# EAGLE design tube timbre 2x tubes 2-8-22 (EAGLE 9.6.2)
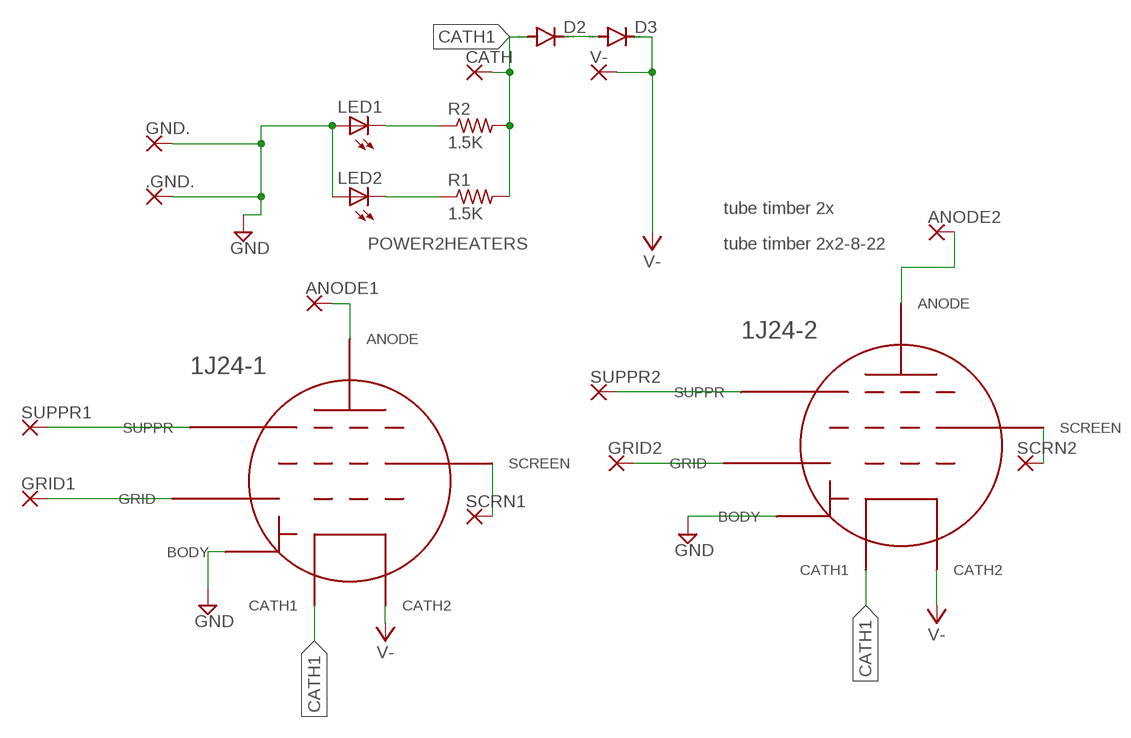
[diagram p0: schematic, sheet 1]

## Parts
1J24-1  1J24B  [6PINSOLDER]
1J24-2  1J24B  [6PINSOLDER]
.GND.  1  WIREPAD1,6/0,9  [1,6/0,9]
ANODE1  1  WIREPAD2,54/1,0  [2,54/1,0]
ANODE2  1  WIREPAD2,54/1,0  [2,54/1,0]
CATH  1  WIREPAD1,6/0,9  [1,6/0,9]
D2  1N4148DO35-7  [DO35-7]
D3  1N4148DO35-7  [DO35-7]
GND.  1  WIREPAD1,6/0,9  [1,6/0,9]
GRID1  1  WIREPAD1,6/0,9  [1,6/0,9]
GRID2  1  WIREPAD1,6/0,9  [1,6/0,9]
LED1  LED3MM  [LED3MM]
LED2  LED3MM  [LED3MM]
R1  1.5K  R-US_0207/10  [0207/10]
R2  1.5K  R-US_0207/10  [0207/10]
SCRN1  1  WIREPAD1,6/0,9  [1,6/0,9]
SCRN2  1  WIREPAD1,6/0,9  [1,6/0,9]
SUPPR1  1  WIREPAD1,6/0,9  [1,6/0,9]
SUPPR2  1  WIREPAD1,6/0,9  [1,6/0,9]
V-  1  WIREPAD1,6/0,9  [1,6/0,9]

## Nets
CATH1: 1J24-1.1-CATH(CATH1) 1J24-2.1-CATH(CATH1) CATH.1(P) D2.A R1.2 R2.2
GND: 1J24-1.3-BDY(BODY) 1J24-2.3-BDY(BODY) .GND..1(P) GND..1(P) LED1.A LED2.A
N$1: 1J24-2.6-GRID(GRID) GRID2.1(P)
N$2: 1J24-1.4-SUPP(SUPPR) SUPPR1.1(P)
N$3: LED2.K(C) R1.1
N$4: 1J24-1.6-GRID(GRID) GRID1.1(P)
N$5: LED1.K(C) R2.1
N$6: 1J24-1.5-SCR(SCREEN) SCRN1.1(P)
N$7: 1J24-2.4-SUPP(SUPPR) SUPPR2.1(P)
N$8: 1J24-1.A(ANODE) ANODE1.1(P)
N$9: D2.C D3.A
N$10: 1J24-2.A(ANODE) ANODE2.1(P)
N$11: 1J24-2.5-SCR(SCREEN) SCRN2.1(P)
V-: 1J24-1.2-CATH(CATH2) 1J24-2.2-CATH(CATH2) D3.C V-.1(P)

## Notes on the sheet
- tube timber 2x
- POWER2HEATERS | tube timber 2x2-8-22

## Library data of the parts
1J24-1 1J24-2 = submini tubes CL:1J24B
.GND. ANODE1 ANODE2 CATH GND. GRID1 GRID2 SCRN1 SCRN2 SUPPR1 SUPPR2 V- = wirepad:WIREPAD: Wire PAD connect wire on PCB; SPICEPREFIX: X
D2 D3 = diode:1N4148: DIODE; SPICEPREFIX: D
LED1 LED2 = adafruit:LED: LED; SPICEPREFIX: L
R1 R2 = resistor:R-US_: RESISTOR, American symbol; SPICEPREFIX: R

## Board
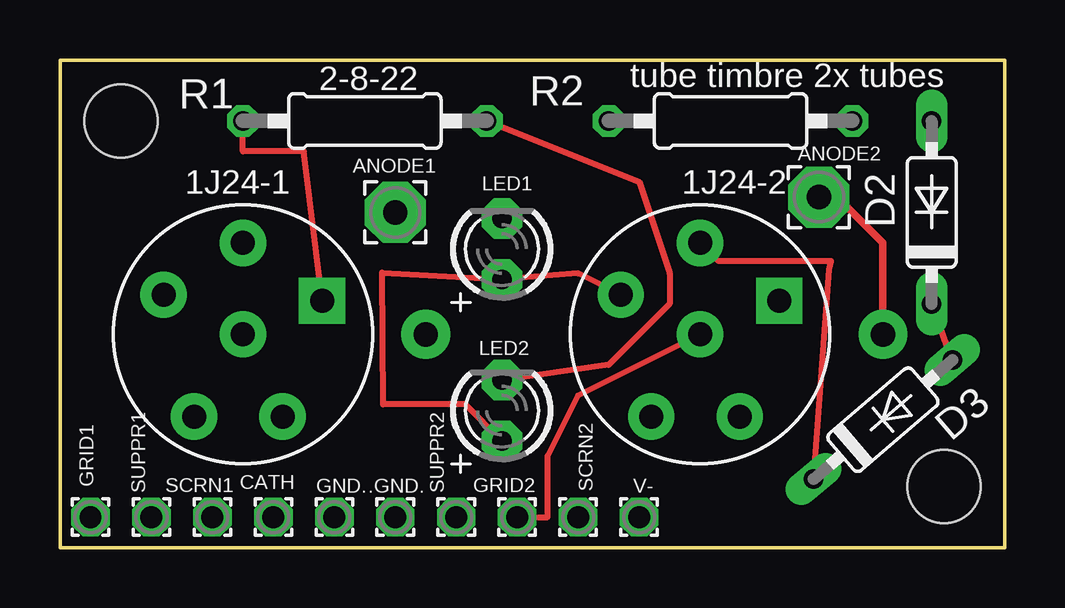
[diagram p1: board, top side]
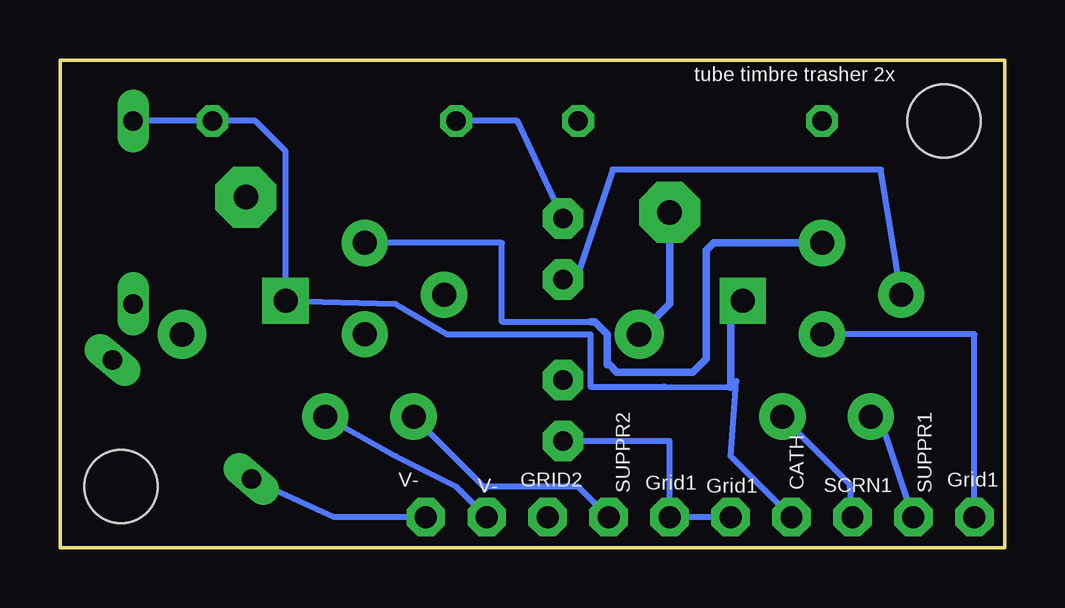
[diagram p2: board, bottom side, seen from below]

Size 39.37 x 20.32 mm. Coordinates in mm from the lower left corner, seen from the top.
Outline: 0,0 0,20.32 39.37,20.32 39.37,0 0,0
Copper layers (1*16): Top 0.035mm / dielectric 1.5mm / Bottom 0.035mm
Design rules "default": minimum track width 6mil, minimum drill 0.35mm, track to track 6mil, track to pad 6mil, pad to pad 6mil, via to via 6mil, smd to smd 6mil, copper to edge 40mil, drill to drill 6mil, minimum pad ring 10mil, minimum via ring 8mil, stop-mask expansion 4mil, vias tented up to drill 0mil, thermal gap 10mil
Holes 3.05 mm at 2.54,17.78 36.83,2.54

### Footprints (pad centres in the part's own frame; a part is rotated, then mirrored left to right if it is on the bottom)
6PINSOLDER = drill 1 pad 1.93 square: 1-CATH 5.842,2.667 | drill 1 pad 1.93: 2-CATH 2.54,5.08; 3-BDY -0.762,2.921; 4-SUPP 0.508,-2.159; 5-SCR 4.191,-2.159; 6-GRID 2.54,1.27 | drill 1.016 pad 2.032: A 10.16,1.27
1,6/0,9 = drill 0.914 pad 1.6 octagon: 1 0,0
2,54/1,0 = drill 1.016 pad 2.54 octagon: 1 0,0
DO35-7 = drill 0.813 long: A 3.81,0; C -3.81,0
LED3MM = drill 0.813 pad 1.676 octagon: A -1.27,0; K 1.27,0
0207/10 = drill 0.813 octagon: 1 -5.08,0; 2 5.08,0

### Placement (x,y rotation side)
1J24-1  5.08,7.62 0 top
1J24-2  24.13,7.62 0 top
.GND.  13.97,1.27 0 top
ANODE1  13.97,13.97 0 top
ANODE2  31.62,14.61 0 top
CATH  8.89,1.27 0 top
D2  36.32,13.97 90 top
D3  34.29,5.33 40.6 top
GND.  11.43,1.27 0 top
GRID1  1.27,1.27 0 top
GRID2  19.05,1.27 0 top
LED1  18.41,12.45 90 top
LED2  18.41,5.71 90 top
R1  12.7,17.78 180 top
R2  27.94,17.78 0 top
SCRN1  6.35,1.27 0 top
SCRN2  21.59,1.27 0 top
SUPPR1  3.81,1.27 0 top
SUPPR2  16.51,1.27 0 top
V-  24.13,1.27 0 top

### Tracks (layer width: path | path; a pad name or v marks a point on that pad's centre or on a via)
CATH1
  Top 0.254: 1J24-1.1-CATH 10.16,16.51 7.62,16.51 R1.2
  Bottom 0.254: D2.A R2.2 31.24,17.78 29.97,16.51 1J24-2.1-CATH 25.4,10.16 23.24,8.89 17.27,8.89 17.27,6.71 14.21,6.71 11.43,6.68 | CATH.1 11.43,3.81 11.19,6.94 11.43,6.94
  Bottom 0.305: 11.43,6.68 11.43,6.94 11.43,9.78 1J24-1.1-CATH
GND
  Top 0.254: 1J24-2.3-BDY 21.59,11.43 LED1.A 13.43,11.46 13.46,5.97 16.89,5.97 LED2.A
  Bottom 0.254: 1J24-1.3-BDY 5.16,15.75 16.34,15.75 17.78,11.43 LED1.A | GND..1 .GND..1 13.97,4.45 LED2.A
N$1
  Top 0.254: GRID2.1 20.32,1.27 20.32,3.81 21.59,6.35 1J24-2.6-GRID
N$2
  Bottom 0.254: SUPPR1.1 5.08,5.08 1J24-1.4-SUPP
N$3
  Top 0.254: R1.1 24.13,15.24 25.4,11.43 25.4,10.16 22.86,7.62 LED2.K
N$4
  Bottom 0.254: GRID1.1 1.27,8.89 1J24-1.6-GRID
N$5
  Bottom 0.254: LED1.K 20.32,17.78 R2.1
N$6
  Bottom 0.254: 1J24-1.5-SCR 6.48,2.67 SCRN1.1
N$7
  Bottom 0.254: SUPPR2.1 17.78,2.54 21.69,2.54 21.65,2.47 1J24-2.4-SUPP
N$8
  Bottom 0.305: 1J24-1.A 13.97,10.16 ANODE1.1
N$9
  Top 0.254: D3.A D2.C
N$10
  Top 0.305: 1J24-2.A 34.29,12.7 32.38,14.61 ANODE2.1
N$11
  Bottom 0.254: SCRN2.1 22.86,2.54 25.4,3.81 1J24-2.5-SCR
V-
  Top 0.254: D3.C 32.04,11.59 32.13,11.94 27.43,11.94 1J24-2.2-CATH
  Bottom 0.254: 17.25,9.42 20.95,9.42 20.95,12.7 1J24-2.2-CATH | V-.1 27.94,1.27 D3.C
  Bottom 0.305: 17.25,9.42 17.09,9.42 16.56,8.89 16.56,7.62 16.47,7.62 16.17,7.32 13.01,7.32 12.45,7.87 12.45,12.39 12.14,12.7 1J24-1.2-CATH

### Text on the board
tNames: 2-8-22 | tube timbre 2x tubes
bNames: tube timbre trasher 2x | Grid1 | SCRN1 | GRID2 | V- | SUPPR1 | CATH | Grid1 | Grid1 | SUPPR2 | V-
